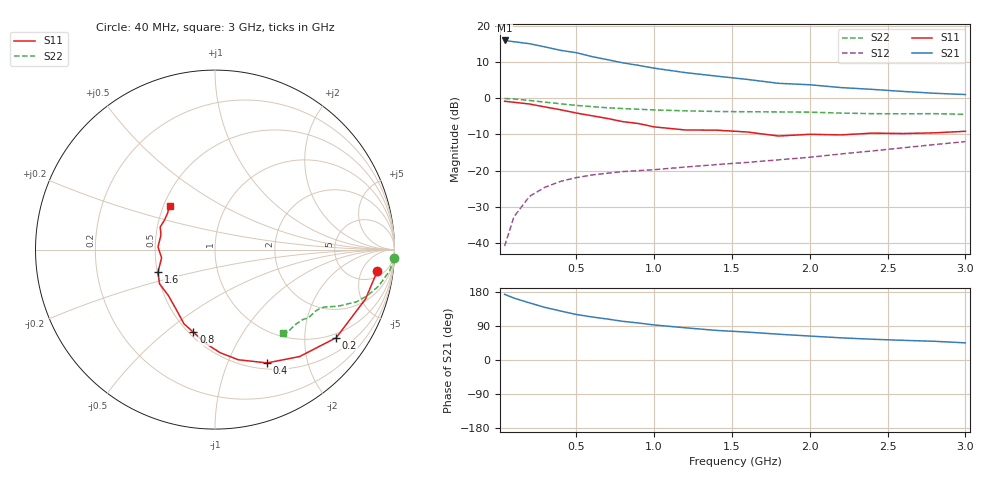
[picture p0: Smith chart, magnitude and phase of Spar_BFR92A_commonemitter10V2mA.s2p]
! Filename:  BFR92AF.S2P  Version:  2.0
! NXP part #: BFR92A  Date: May 1990
! Bias condition: Vce=10V, Ic=2mA
#  MHz  S  MA  R  50
! Freq  S11  S21  S12  S22  !GUM [dB]
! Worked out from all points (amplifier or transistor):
!   21 points, 40 MHz to 3 GHz, reference 50 ohm
!   highest |S21| = 16.0 dB at 40 MHz (marker M1)
!   |S21| within 3 dB of that: start of sweep to 440.6 MHz
!   unconditionally stable (mu >= 1): 1.612 GHz to 2.75 GHz
!   at 300 MHz: K = 0.29, MSG = 19.4 dB, |S12| = -24.6 dB
!   at 1 GHz: K = 0.82, MSG = 14.0 dB, |S12| = -19.7 dB
!   at 3 GHz: K = 0.96, MSG = 6.5 dB, |S12| = -12.0 dB
!   S11 on the Smith chart (normalised r, x): 40 MHz: 7, -10; 200 MHz: 0.87, -2.84; 400 MHz: 0.57, -1.40; 800 MHz: 0.53, -0.63; 1.6 GHz: 0.50, -0.14; 3 GHz: 0.54, +0.30
40  0.912 -7.6  6.327 173.3  0.009 85.6  0.996 -2.7
100  0.883 -18.1  6.077 163.4  0.023 79.1  0.981 -6.8
200  0.835 -36.0  5.703 150.7  0.044 71.0  0.935 -12.5
300  0.76 -51.6  5.148 138.7  0.059 64.1  0.886 -16.9
400  0.695 -65.3  4.614 129.3  0.071 59.3  0.84 -20.3
500  0.627 -78.1  4.289 120.2  0.08 56.3  0.798 -22.3
600  0.575 -87.2  3.789 113.7  0.087 54.4  0.769 -23.9
700  0.527 -95.3  3.431 108.1  0.092 54.1  0.741 -25.3
800  0.476 -104.7  3.099 102.1  0.097 53.3  0.722 -26.1
900  0.448 -112.7  2.861 97.6  0.1 54.5  0.707 -26.9
1000  0.403 -121.5  2.617 92.5  0.103 55.1  0.691 -27.5
1200  0.365 -135.2  2.272 85.0  0.112 57.4  0.672 -29.1
1400  0.363 -148.4  2.033 78.1  0.121 59.6  0.658 -31.1
1600  0.342 -158.3  1.827 73.6  0.13 64.0  0.653 -32.5
1800  0.301 -171.2  1.614 68.1  0.141 67.3  0.649 -34.4
2000  0.318 177.4  1.542 63.2  0.153 70.0  0.644 -36.2
2200  0.312 164.9  1.41 58.5  0.17 73.0  0.625 -38.6
2400  0.33 157.6  1.332 54.8  0.187 74.2  0.614 -42.2
2600  0.326 150.0  1.246 51.9  0.207 75.2  0.611 -45.9
2800  0.333 142.6  1.176 49.4  0.229 76.7  0.614 -48.6
3000  0.35 136.4  1.129 45.2  0.252 76.5  0.601 -50.6
